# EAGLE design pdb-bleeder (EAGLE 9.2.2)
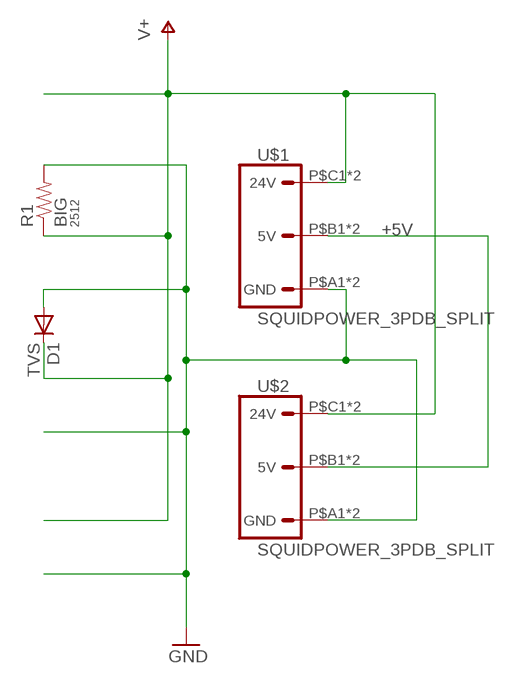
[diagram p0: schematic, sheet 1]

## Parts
D1  TVS  DIODESMA403D  [SMA-403D]
R1  BIG  RESISTOR2512  [R2512]
U$1  SQUIDPOWER_3PDB_SPLIT  [PDBCONN_ABC]
U$2  SQUIDPOWER_3PDB_SPLIT  [PDBCONN_ABC]

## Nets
+5V: U$1.P$B1(5V) U$1.P$B2(5V) U$2.P$B1(5V) U$2.P$B2(5V)
GND: D1.P$2(A) R1.2 U$1.P$A1(GND) U$1.P$A2(GND) U$2.P$A1(GND) U$2.P$A2(GND)
V+: D1.P$1(C) R1.1 U$1.P$C1(24V) U$1.P$C2(24V) U$2.P$C1(24V) U$2.P$C2(24V)

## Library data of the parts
D1 = passives:DIODE: DIODE
R1 = passives:RESISTOR: Resistor; PACKAGE: 2512
U$1 U$2 = connector:SQUIDPOWER_3

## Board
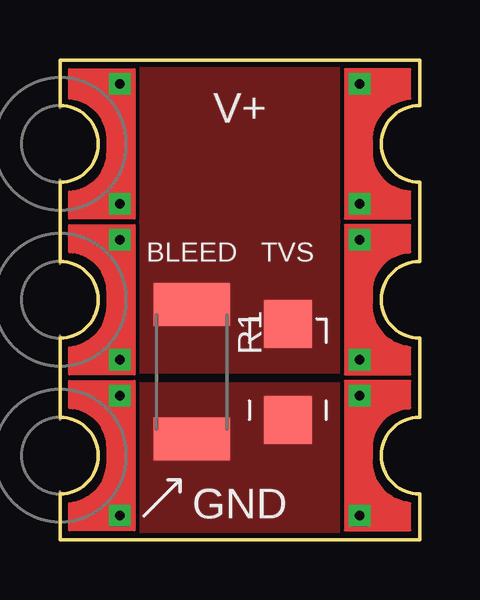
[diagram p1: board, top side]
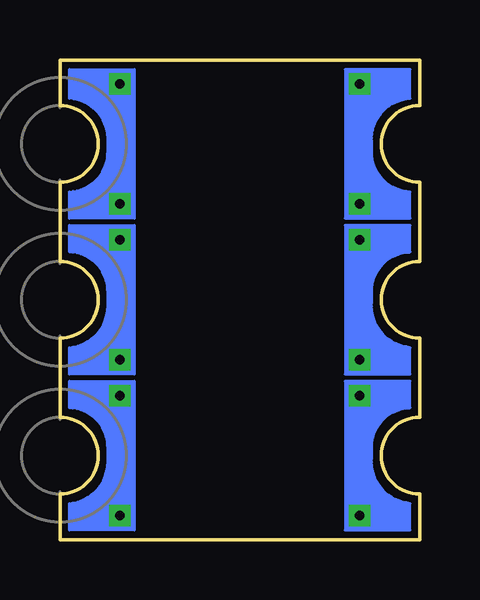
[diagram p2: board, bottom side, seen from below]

Size 15 x 20 mm. Coordinates in mm from the lower left corner, seen from the top.
Outline: 0,5.1 0,8.4 arc90 1.6,10 arc90 0,11.6 0,14.9 arc90 1.6,16.5 arc90 0,18.1 0,20 15,20 15,18.1 arc90 13.4,16.5 arc90 15,14.9 15,11.6 arc90 13.4,10 arc90 15,8.4 15,5.1 arc90 13.4,3.5 arc90 15,1.9 15,0 0,0 0,1.9 arc90 1.6,3.5 arc90 0,5.1
Copper layers (1*16): Top 0.035mm / dielectric 1.5mm / Bottom 0.035mm
Design rules "default *": minimum track width 6mil, minimum drill 0.35mm, track to track 6mil, track to pad 6mil, pad to pad 6mil, via to via 6mil, smd to smd 6mil, copper to edge 8mil, drill to drill 6mil, minimum pad ring 10mil, minimum via ring 8mil, stop-mask expansion 4mil, vias tented up to drill 0mil, thermal gap 10mil

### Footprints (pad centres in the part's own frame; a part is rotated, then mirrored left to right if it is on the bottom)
SMA-403D = smd 2 x 2: P$1 -2,0; P$2 2,0
R2512 = smd 1.8 x 3.2: 1 -2.8,0; 2 2.8,0
PDBCONN_ABC = drill 0.4 square: P$A1 2.5,-9; P$A2 2.5,-4; P$B1 2.5,-2.5; P$B2 2.5,2.5; P$C1 2.5,4; P$C2 2.5,9

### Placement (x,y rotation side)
D1  9.5,7 270 top
R1  5.5,7 270 top
U$1  15,10 0 bottom
U$2  0,10 0 top

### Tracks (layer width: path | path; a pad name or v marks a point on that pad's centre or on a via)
+5V
  pour Bottom (no thermals): -1.5,13 18,13 18,7 -1.5,7
GND
  pour Top (no thermals): -1,6.5 17.5,6.5 17.5,-0.5 -1,-0.5
  pour Bottom (no thermals): -1.5,6.5 18,6.5 18,-1 -1.5,-1
V+
  pour Top (no thermals): -1,7 17.5,7 17.5,20.5 -1,20.5
  pour Bottom (no thermals): -1.5,13.5 18,13.5 18,21 -1.5,21

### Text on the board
tPlace: V+ | BLEED | TVS | GND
